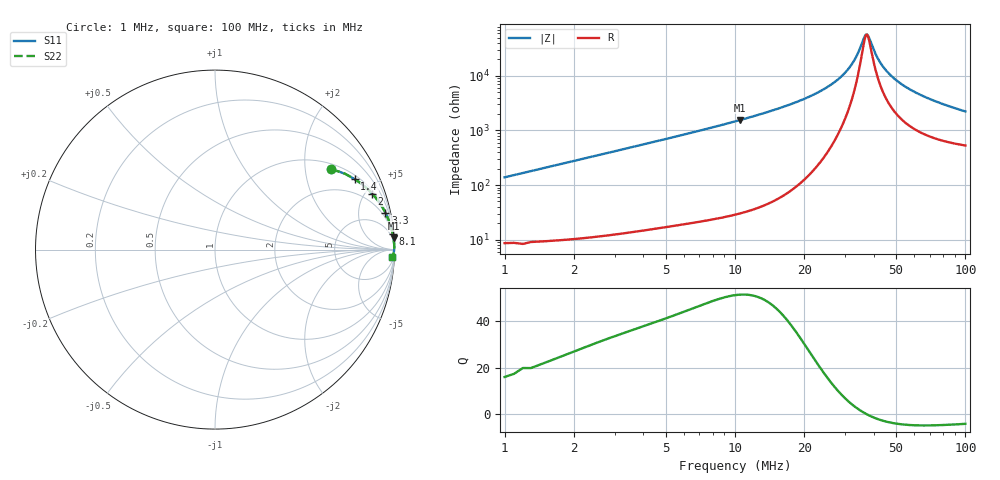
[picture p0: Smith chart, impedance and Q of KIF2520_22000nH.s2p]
!version-2
!date-12.2020
!Series
# MHz S RI R 50
!Freq ReS11 ImS11 ReS21 ImS21 ReS12 ImS12 ReS22 ImS22
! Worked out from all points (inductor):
!   991 points, 1 MHz to 100 MHz, reference 50 ohm
!   read as one part in series: L = 21.9 uH near 1.4 MHz
!   highest Q = 51.4 at 10.5 MHz (marker M1), where L = 23.5 uH
!   self-resonance near 37.3 MHz
!   S11 on the Smith chart (normalised r, x): 1 MHz: 1.17, +2.76; 1.4 MHz: 1.18, +3.87; 2 MHz: 1.20, +5.53; 3.3 MHz: 1.26, +9.13; 8.1 MHz: 1, +23; 100 MHz: 12, -43
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1  0.6483 0.4474  0.3517 -0.4474  0.3517 -0.4474  0.6483 0.4474
1.4  0.7787 0.3921  0.2213 -0.3921  0.2213 -0.3921  0.7787 0.3921
2  0.8755 0.3122  0.1245 -0.3122  0.1245 -0.3122  0.8755 0.3122
3.3  0.9489 0.2063  0.0511 -0.2063  0.0511 -0.2063  0.9489 0.2063
5.3  0.979 0.132  0.021 -0.132  0.021 -0.132  0.979 0.132
8.1  0.9909 0.0855  0.00914 -0.0855  0.00914 -0.0855  0.9909 0.0855
10.5  0.9946 0.0641  0.00539 -0.0641  0.00539 -0.0641  0.9946 0.0641
17.5  0.9981 0.0328  0.00193 -0.0328  0.00193 -0.0328  0.9981 0.0328
28.2  0.9987 0.0112  0.00128 -0.0112  0.00128 -0.0112  0.9987 0.0112
31.5  0.9986 0.00674  0.00138 -0.00674  0.00138 -0.00674  0.9986 0.00674
34  0.9985 0.00371  0.00151 -0.00371  0.00151 -0.00371  0.9985 0.00371
36.4  0.9983 0.00103  0.00167 -0.00103  0.00167 -0.00103  0.9983 0.00103
37.4  0.9983 -3.72e-05  0.00174 3.72e-05  0.00174 3.72e-05  0.9983 -3.72e-05
38.1  0.9982 -0.000763  0.0018 0.000763  0.0018 0.000763  0.9982 -0.000763
40.9  0.998 -0.00354  0.00204 0.00354  0.00204 0.00354  0.998 -0.00354
43  0.9978 -0.0055  0.00224 0.0055  0.00224 0.0055  0.9978 -0.0055
46.3  0.9974 -0.00842  0.00259 0.00842  0.00259 0.00842  0.9974 -0.00842
50.5  0.9969 -0.0119  0.00309 0.0119  0.00309 0.0119  0.9969 -0.0119
57.6  0.9959 -0.0173  0.00405 0.0173  0.00405 0.0173  0.9959 -0.0173
67  0.9945 -0.0237  0.00554 0.0237  0.00554 0.0237  0.9945 -0.0237
83.5  0.9913 -0.0337  0.00867 0.0337  0.00867 0.0337  0.9913 -0.0337
100  0.9876 -0.0425  0.0124 0.0425  0.0124 0.0425  0.9876 -0.0425
